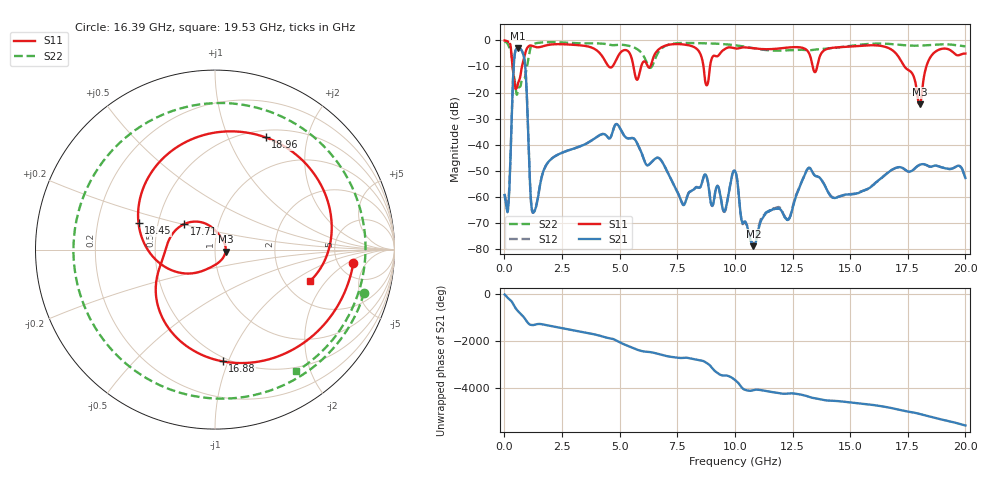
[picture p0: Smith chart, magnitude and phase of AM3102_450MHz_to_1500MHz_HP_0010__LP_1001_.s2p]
!Agilent Technologies,E8364B,MY43040894,A.07.50.67
!Agilent E8364B: A.07.50.67
!Date: Thursday, January 11, 2018 05:28:00
!Correction: S11(Full 2 Port(1,2))
!S21(Full 2 Port(1,2))
!S12(Full 2 Port(1,2))
!S22(Full 2 Port(1,2))
!S2P File: Measurements: S11, S21, S12, S22:
# Hz S  dB  R 50
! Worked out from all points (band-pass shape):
!   1601 points, 10 MHz to 20 GHz, reference 50 ohm
!   highest |S21| = -3.00 dB at 584.7 MHz (marker M1); lowest = -78.9 dB at 10.8 GHz (marker M2)
!   |S21| within 3 dB of the highest: 441.3 MHz to 837.1 MHz (395.7 MHz wide, 61.9 % of centre)
!   lowest |S11| = -24.5 dB at 18.01 GHz (marker M3), VSWR 1.13, Z = 56.2 - j1.28 ohm
!   |S11| at or under -10 dB: 355.5 MHz to 763.2 MHz (407.7 MHz wide, 72.9 % of centre); 5.6 GHz to 5.934 GHz (333.4 MHz wide, 5.78 % of centre); 17.35 GHz to 18.31 GHz (952.5 MHz wide, 5.34 % of centre)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
!   |S22| runs from -20.9 to -0.4 dB; largest |S21 - S12| = 0.0012
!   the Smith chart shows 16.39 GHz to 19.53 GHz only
!   S11 on the Smith chart (normalised r, x): 16.39 GHz: 6.93, -2.54; 16.88 GHz: 0.47, -0.95; 17.71 GHz: 0.68, +0.20; 18.45 GHz: 0.39, +0.14; 18.96 GHz: 0.58, +1.38; 19.53 GHz: 2.75, -1.39
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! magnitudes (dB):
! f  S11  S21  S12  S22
! 10 MHz  0.0  -59.3  -58.9  -0.4
! 172.4 MHz  -0.6  -63.6  -62.3  -1.9
! 409.8 MHz  -14.3  -9.2  -9.2  -13.4
! 584.7 MHz  -16.7  -3.0  -3.0  -19.0
! 884.6 MHz  -5.7  -8.3  -8.3  -14.4
! 1.259 GHz  -2.3  -66.0  -66.0  -1.4
! 3.346 GHz  -2.0  -40.4  -40.4  -1.1
! 6.682 GHz  -3.6  -45.1  -45.0  -4.6
! 7.756 GHz  -1.6  -63.1  -63.0  -1.0
! 8.781 GHz  -17.3  -52.5  -52.4  -1.2
! 10.01 GHz  -3.1  -50.1  -50.1  -1.9
! 10.8 GHz  -3.0  -78.9  -78.2  -3.0
! 13.34 GHz  -8.6  -50.1  -50.1  -3.7
! 16.39 GHz  -2.2  -52.5  -52.6  -1.3
! 16.68 GHz  -3.0  -50.5  -50.4  -1.4
! 16.88 GHz  -4.1  -49.3  -49.3  -1.5
! 17.71 GHz  -13.0  -49.8  -49.8  -2.1
! 18.01 GHz  -24.5  -47.8  -47.7  -2.0
! 18.45 GHz  -6.9  -48.4  -48.4  -1.8
! 18.96 GHz  -3.3  -48.7  -48.7  -1.5
! 19.53 GHz  -5.1  -48.8  -48.7  -1.8
! 20 GHz  -5.1  -52.8  -52.6  -2.3
